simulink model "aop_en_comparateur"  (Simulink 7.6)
settings: Solver=ode15s  StartTime=0.0  StopTime=0.01  RelTol=1e-3
StopFcn:
  | close all, clc
  | load signaux.mat
  | plotyy(x(1,:),x(2,:),x(1,:),x(3,:))
  | title('Amplificateur opérationnel en comparateur')
  | xlabel('temps')
  | grid
libraries: fl_lib x7, nesl_utility x3, elec_lib x1

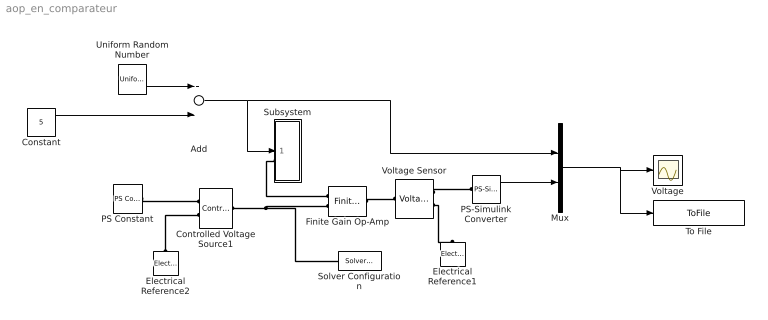
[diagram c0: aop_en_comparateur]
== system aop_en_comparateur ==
  Add : Sum
  Constant : Constant  Value=5
  Controlled Voltage Source1 : fl_lib/Electrical/Electrical Sources/Controlled Voltage Source  DialogController=NetworkEngine.DynNeDlgSource  SystemSampleTime=-1  i_Log=off  v_Log=off  LocalVarNames=|current|voltage|power  LocalVarDescs=|Current (A)|Voltage (V)|Power (W)  LocalVarLogging=[0 0 0]
  Electrical Reference1 : fl_lib/Electrical/Electrical Elements/Electrical Reference  DialogController=NetworkEngine.DynNeDlgSource  SystemSampleTime=-1  i_Log=off  LocalVarNames=|i  LocalVarDescs=|i  LocalVarLogging=[]
  Electrical Reference2 : fl_lib/Electrical/Electrical Elements/Electrical Reference  DialogController=NetworkEngine.DynNeDlgSource  SystemSampleTime=-1  i_Log=off  LocalVarNames=|i  LocalVarDescs=|i  LocalVarLogging=[]
  Finite Gain Op-Amp : elec_lib/Integrated Circuits/Finite Gain Op-Amp  DialogController=NetworkEngine.DynNeDlgSource  SystemSampleTime=-1  A=1000  Rin=1e+06 Ohm  Rout=100 Ohm  Vmin=-15 V  Vmax=15 V  LocalVarNames=|power  LocalVarDescs=|Dissipated power (W)  LocalVarLogging=0
  Mux : Mux  Inputs=2
  PS Constant : fl_lib/Physical Signals/Sources/PS Constant  DialogController=NetworkEngine.DynNeDlgSource  SystemSampleTime=-1  constant=5  LocalVarLogging=[]
  PS-Simulink Converter : nesl_utility/PS-Simulink Converter  DialogController=NetworkEngine.DynNeUtilDlgSource  SystemSampleTime=-1  PhysicalDomain=network_engine_domain  LeftPortType=input  RightPortType=output  SubClassName=ps_output  Unit=1  AffineConversion=off
  Solver Configuration : nesl_utility/Solver Configuration  DialogController=NetworkEngine.DynNeUtilDlgSource  SystemSampleTime=-1  PhysicalDomain=network_engine_domain  LeftPortType=input  RightPortType=generic  SubClassName=solver  Accelerate=off  Profile=off  ResidualTolerance=1e-9  MaxNonlinIter=12  MaxModeIter=2  DoFixedCost=off  UseLocalSampling=off  DoDC=off  LinearAlgebra=Sparse  LocalSolverSampleTime=.001  LocalSolverChoice=NE_BACKWARD_EULER_ADVANCER  UseLocalSolver=off
  Subsystem : Subsystem
  To File : ToFile  Filename=signaux  MatrixName=x
  Uniform Random Number : UniformRandomNumber
  Voltage : Scope
  Voltage Sensor : fl_lib/Electrical/Electrical Sensors/Voltage Sensor  DialogController=NetworkEngine.DynNeDlgSource  SystemSampleTime=-1  i1_Log=off  v1_Log=off  LocalVarNames=|i1|v1  LocalVarDescs=|i1|v1  LocalVarLogging=[]
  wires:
  Mux/1 -> To File/1, Voltage/1
  PS-Simulink Converter/1 -> Mux/2
  Uniform Random Number/1 -> Add/1
  Constant/1 -> Add/2
  Add/1 -> Subsystem/1(S), Mux/1
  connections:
  Electrical Reference2/LConn1 -- Controlled Voltage Source1/RConn2
  Voltage Sensor/RConn1 -- PS-Simulink Converter/LConn1
  Voltage Sensor/RConn2 -- Electrical Reference1/LConn1
  PS Constant/RConn1 -- Controlled Voltage Source1/RConn1
  Controlled Voltage Source1/LConn1 -- Finite Gain Op-Amp/LConn2 -- Solver Configuration/RConn1
  Finite Gain Op-Amp/RConn1 -- Voltage Sensor/LConn1
  Subsystem/LConn1 -- Finite Gain Op-Amp/LConn1

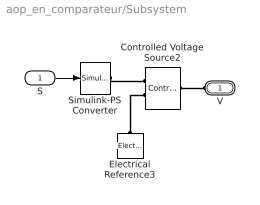
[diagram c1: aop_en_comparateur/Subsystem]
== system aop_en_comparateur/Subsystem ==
  S : Inport
  Controlled Voltage Source2 : fl_lib/Electrical/Electrical Sources/Controlled Voltage Source  DialogController=NetworkEngine.DynNeDlgSource  SystemSampleTime=-1  i_Log=off  v_Log=off  LocalVarNames=|current|voltage|power  LocalVarDescs=|Current (A)|Voltage (V)|Power (W)  LocalVarLogging=[0 0 0]
  Electrical Reference3 : fl_lib/Electrical/Electrical Elements/Electrical Reference  DialogController=NetworkEngine.DynNeDlgSource  SystemSampleTime=-1  i_Log=off  LocalVarNames=|i  LocalVarDescs=|i  LocalVarLogging=[]
  Simulink-PS Converter : nesl_utility/Simulink-PS Converter  DialogController=NetworkEngine.DynNeUtilDlgSource  SystemSampleTime=-1  PhysicalDomain=network_engine_domain  LeftPortType=input  RightPortType=output  SubClassName=ps_input  Unit=1  AffineConversion=off  InputFilterTimeConstant=.001  UdotUserProvided=0
  V : PMIOPort  Port=1  Side=Left
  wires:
  S/1 -> Simulink-PS Converter/1
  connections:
  Simulink-PS Converter/RConn1 -- Controlled Voltage Source2/RConn1
  Electrical Reference3/LConn1 -- Controlled Voltage Source2/RConn2
  V/RConn1 -- Controlled Voltage Source2/LConn1
